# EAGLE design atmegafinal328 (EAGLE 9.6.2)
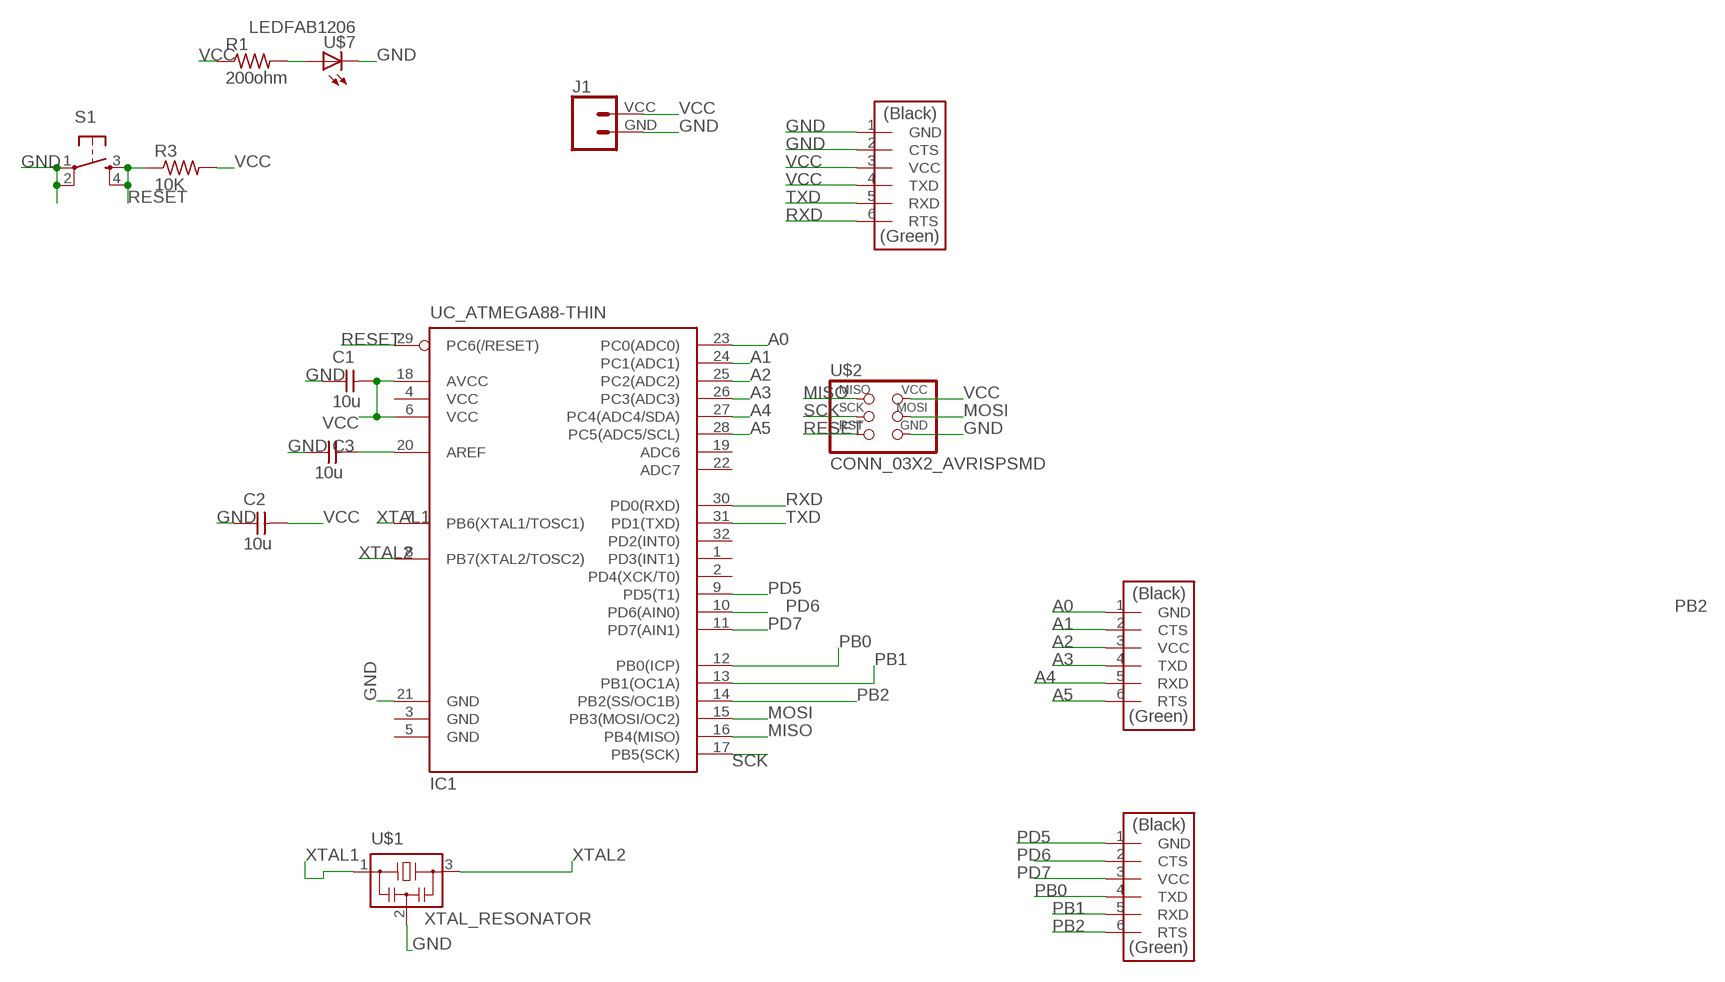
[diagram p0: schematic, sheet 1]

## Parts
C1  10u  CAP_UNPOLARIZEDFAB  [C1206FAB]
C2  10u  CAP_UNPOLARIZEDFAB  [C1206FAB]
C3  10u  CAP_UNPOLARIZEDFAB  [C1206FAB]
IC1  UC_ATMEGA88-THIN  [TQFP32-08THIN]
J1  CONN_024UCON-15767  [JST-2-SMD-VERT]
R1  200ohm  R1206FAB  [R1206FAB]
R3  10K  R1206FAB  [R1206FAB]
S1  SW_SWITCH_TACTILE_6MM6MM_SWITCH  [6MM_SWITCH]
U$1  XTAL_RESONATOR  [EFOBM]
U$2  CONN_03X2_AVRISPSMD  [2X03SMD]
U$3  CONN_06_FTDI-SMD-HEADER  [1X06SMD]
U$4  CONN_06_FTDI-SMD-HEADER  [1X06SMD]
U$6  CONN_06_FTDI-SMD-HEADER  [1X06SMD]
U$7  LEDFAB1206  [LED1206FAB]

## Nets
A0: IC1.23(PC0(ADC0)) U$4.1(GND)
A1: IC1.24(PC1(ADC1)) U$4.2(CTS)
A2: IC1.25(PC2(ADC2)) U$4.3(VCC)
A3: IC1.26(PC3(ADC3)) U$4.4(TXD)
A4: IC1.27(PC4(ADC4/SDA)) U$4.5(RXD)
A5: IC1.28(PC5(ADC5/SCL)) U$4.6(RTS)
GND: C1.1 C2.1 C3.1 IC1.21(GND) J1.GND S1.1(P) S1.2(P1) U$1.2 U$2.6(GND) U$3.1(GND) U$3.2(CTS) U$7.2(C)
MISO: IC1.16(PB4(MISO)) U$2.1(MISO)
MOSI: IC1.15(PB3(MOSI/OC2)) U$2.4(MOSI)
N$1: R1.2 U$7.1(A)
N$2: C3.2 IC1.20(AREF)
PB0: IC1.12(PB0(ICP)) U$6.4(TXD)
PB1: IC1.13(PB1(OC1A)) U$6.5(RXD)
PB2: IC1.14(PB2(SS/OC1B)) U$6.6(RTS)
PD5: IC1.9(PD5(T1)) U$6.1(GND)
PD6: IC1.10(PD6(AIN0)) U$6.2(CTS)
PD7: IC1.11(PD7(AIN1)) U$6.3(VCC)
RESET: IC1.29(PC6(/RESET)) R3.1 S1.3(S) S1.4(S1) U$2.5(RST)
RXD: IC1.30(PD0(RXD)) U$3.6(RTS)
SCK: IC1.17(PB5(SCK)) U$2.3(SCK)
TXD: IC1.31(PD1(TXD)) U$3.5(RXD)
VCC: C1.2 C2.2 IC1.6(VCC) IC1.18(AVCC) J1.VCC R1.1 R3.2 U$2.2(VCC) U$3.3(VCC) U$3.4(TXD)
XTAL1: IC1.7(PB6(XTAL1/TOSC1)) U$1.1
XTAL2: IC1.8(PB7(XTAL2/TOSC2)) U$1.3
Unconnected: IC1.1(PD3(INT1)) IC1.2(PD4(XCK/T0)) IC1.19(ADC6) IC1.22(ADC7) IC1.32(PD2(INT0))

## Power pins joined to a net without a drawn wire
GND: IC1.3(GND) IC1.5(GND)
VCC: IC1.4(VCC)

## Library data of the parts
C1-C3 = fab:CAP_UNPOLARIZED
IC1 = fab:UC_ATMEGA88-THIN
J1 = SparkFun-Connectors:CONN_02: Multi connection point. Often used as Generic Header-pin footprint for 0.1 inch spaced/style header connections
R1 R3 = fab:R: Resistor (US Symbol)
S1 = fab:SW_SWITCH_TACTILE_6MM: OMRON SWITCH
U$1 = fab:XTAL_RESONATOR
U$2 = fab:CONN_03X2_AVRISP
U$3 U$4 U$6 = fab:CONN_06_FTDI-SMD-HEADER
U$7 = fab:LED: LED

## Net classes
0 default: width 0.305 mm, drill 0.356 mm, clearance 0.305 mm

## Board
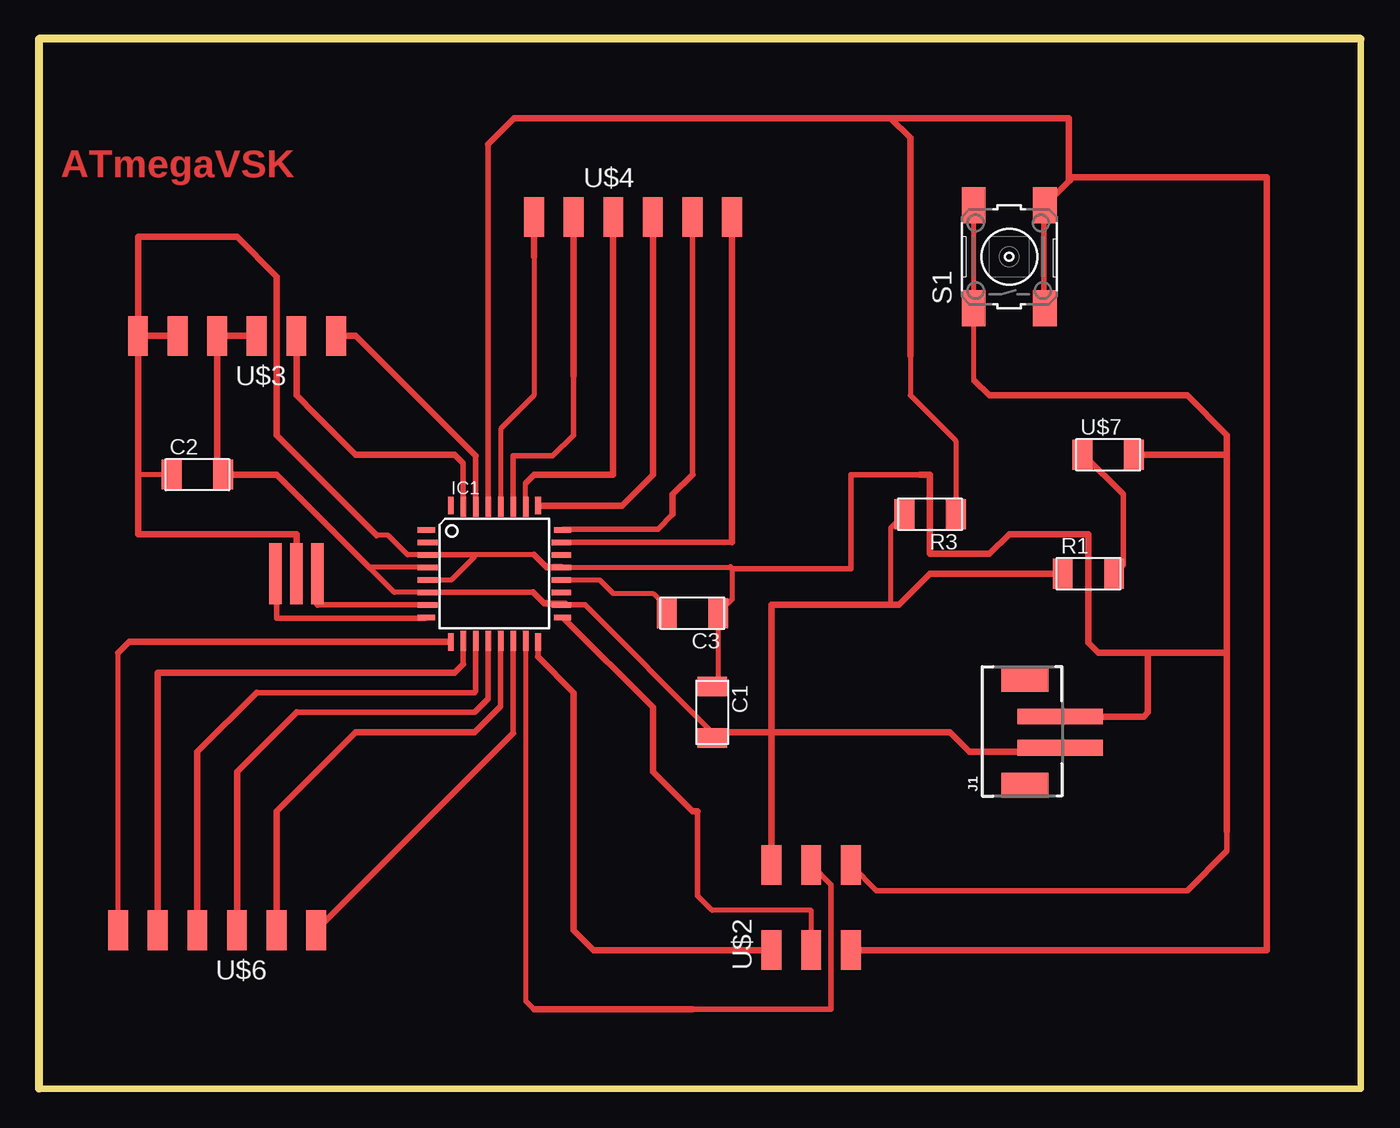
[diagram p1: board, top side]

Size 84.76 x 67.3 mm. Coordinates in mm from the lower left corner, seen from the top.
Outline: 0,67.3 0,0 84.76,0 84.76,67.3 0,67.3
Copper layers (1*16): Top 0.035mm / dielectric 1.5mm / Bottom 0.035mm
Design rules "default *": minimum track width 12mil, minimum drill 0.35mm, track to track 14mil, track to pad 14mil, pad to pad 6mil, via to via 6mil, smd to smd 6mil, copper to edge 40mil, drill to drill 6mil, minimum pad ring 10mil, minimum via ring 8mil, stop-mask expansion 4mil, vias tented up to drill 0mil, thermal gap 10mil

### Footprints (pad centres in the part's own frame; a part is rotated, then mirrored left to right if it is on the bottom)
C1206FAB = smd 1.27 x 1.905: 1 -1.651,0; 2 1.651,0
TQFP32-08THIN = smd 1.118 x 0.356: 1 -4.369,2.8; 8 -4.369,-2.8; 17 4.369,-2.8; 24 4.369,2.8 | smd 1.27 x 0.356: 2 -4.293,2; 3 -4.293,1.2; 4 -4.293,0.4; 5 -4.293,-0.4; 6 -4.293,-1.2; 7 -4.293,-2; 18 4.293,-2; 19 4.293,-1.2; 20 4.293,-0.4; 21 4.293,0.4; 22 4.293,1.2; 23 4.293,2 | smd 0.356 x 1.118: 9 -2.8,-4.369; 16 2.8,-4.369; 25 2.8,4.369; 32 -2.8,4.369 | smd 0.356 x 1.27: 10 -2,-4.293; 14 1.2,-4.293; 15 2,-4.293; 26 2,4.293; 27 1.2,4.293; 31 -2,4.293 | smd 0.35 x 1.27: 11 -1.2,-4.293; 12 -0.4,-4.293; 13 0.4,-4.293; 28 0.4,4.293; 29 -0.4,4.293; 30 -1.2,4.293
JST-2-SMD-VERT = smd 1 x 5.5: GND 1,-2; VCC -1,-2 | smd 1.6 x 3: P$1 -3.4,0.27; P$2 3.4,0.27
R1206FAB = smd 1.27 x 1.905: 1 -1.651,0; 2 1.651,0
6MM_SWITCH = smd 2.286 x 1.524: 1 -3.302,2.286; 2 3.302,2.286; 3 -3.302,-2.286; 4 3.302,-2.286
EFOBM = smd 0.8 x 3.9: 1 -1.35,0; 2 0,0; 3 1.35,0
2X03SMD = smd 2.54 x 1.27: 1 -2.54,2.54; 2 2.92,2.54; 3 -2.54,0; 4 2.92,0; 5 -2.54,-2.54; 6 2.92,-2.54
1X06SMD = smd 2.54 x 1.27: 1 0,6.35; 2 0,3.81; 3 0,1.27; 4 0,-1.27; 5 0,-3.81; 6 0,-6.35
LED1206FAB = smd 1.27 x 1.905: 1 -1.651,0; 2 1.651,0

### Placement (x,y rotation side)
C1  43.18,24.13 270 top
C2  10.16,39.37 0 top
C3  41.91,30.48 180 top
IC1  29.21,33.02 0 top
J1  63.5,22.86 90 top
R1  67.31,33.02 0 top
R3  57.15,36.83 180 top
S1  62.23,53.34 90 top
U$1  16.51,33.02 180 top
U$2  49.53,11.43 90 top
U$3  12.7,48.26 90 top
U$4  38.1,55.88 270 top
U$6  11.43,10.16 90 top
U$7  68.58,40.64 0 top

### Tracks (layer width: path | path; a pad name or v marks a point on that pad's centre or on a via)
A0
  Top 0.356: IC1.23 44.45,35.02
  Top 0.406: U$4.1 44.45,35.02
A1
  Top 0.356: IC1.24 33.66,35.88 39.69,35.88 40.64,36.83 | U$4.2 41.91,39.37
  Top 0.406: 40.64,36.83 40.64,38.1 41.91,39.37
A2
  Top 0.406: U$4.3 39.37,39.37 37.39,37.39 IC1.25
A3
  Top 0.305: IC1.26 31.21,38.83
  Top 0.356: 31.21,38.83 31.75,39.37
  Top 0.406: 31.75,39.37 36.83,39.37 U$4.4
A4
  Top 0.356: IC1.27 30.41,40.57 32.95,40.57 34.29,41.91 34.29,45.72
  Top 0.406: U$4.5 34.29,45.72
A5
  Top 0.305: U$4.6 31.7,55.68 31.7,54.69 31.75,54.61 | 31.75,53.34 31.75,44.45 29.61,42.31 IC1.28
  Top 0.406: 31.75,54.61 31.75,53.34
GND
  Top 0.305: 60.01,45.4 59.94,45.47 S1.1 S1.2 | IC1.3 23.65,34.22 22.38,35.49 21.66,35.49 | IC1.5 26.46,32.62 27.91,34.07 27.77,34.22 IC1.3 | 44.45,33.34 44.45,31.37 C3.1 43.56,26.16 C1.1 | 31.75,34.22 IC1.3 | U$2.6 53.72,12.7 | C2.1 6.35,39.37 | IC1.21 44.37,33.42
  Top 0.356: 70.17,40.64 U$7.2 | 44.45,33.34 52.07,33.34 52.07,39.37 56.52,39.37 | 53.72,12.7 73.66,12.7 76.2,15.24 76.2,16.51
  Top 0.406: 60.01,45.4 60.96,44.45 73.66,44.45 76.2,41.91 76.2,40.64 | 76.2,40.64 76.2,27.94 | 76.2,27.94 76.2,16.51 | 70.17,40.64 76.2,40.64 | 71.12,27.94 67.94,27.94 67.31,28.58 67.31,35.56 62.23,35.56 60.96,34.29 57.15,34.29 57.15,39.37 56.52,39.37 | 71.12,27.94 76.2,27.94 | U$3.1 6.35,54.61 12.7,54.61 15.24,52.07 15.24,41.91 21.66,35.49 | U$1.2 16.51,35.56 6.35,35.56 6.35,39.37 U$3.1 | 44.37,33.42 44.45,33.34 | IC1.21 32.55,33.42 31.75,34.22 | U$3.1 U$3.2 | J1.GND 70.85,23.86 71.12,24.13 71.12,27.94
MISO
  Top 0.356: IC1.16 32.01,27.68
  Top 0.406: 32.01,27.68 34.29,25.4 34.29,10.16 35.56,8.89 U$2.1
MOSI
  Top 0.305: IC1.15 31.24,28.7 31.24,5.59 31.75,5.08
  Top 0.356: 41.91,5.08 50.8,5.08 50.8,13.08 U$2.4
  Top 0.406: 41.91,5.08 31.75,5.08
N$1
  Top 0.356: R1.2 69.53,33.59 69.53,38.1 66.99,40.64 U$7.1
N$2
  Top 0.305: IC1.20 35.96,32.62 36.83,31.75 39.37,31.75 40.26,30.86 C3.2
PB0
  Top 0.356: IC1.12 28.81,25 27.94,24.13 16.51,24.13
  Top 0.406: 16.51,24.13 12.7,20.32 U$6.4
PB1
  Top 0.356: 27.94,22.86 29.61,24.53 IC1.13
  Top 0.406: 27.94,22.86 20.32,22.86 15.24,17.78 U$6.5
PB2
  Top 0.356: IC1.14 30.41,22.79
  Top 0.406: 30.41,22.79 U$6.6
PD5
  Top 0.305: U$6.1 5.08,27.94
  Top 0.406: IC1.9 5.79,28.65 5.08,27.94
PD6
  Top 0.356: IC1.10 27.21,27.21
  Top 0.406: 27.21,27.21 26.67,26.67 7.62,26.67 U$6.2
PD7
  Top 0.356: 13.97,25.4 27.94,25.4 28.01,25.47 IC1.11
  Top 0.406: U$6.3 10.16,21.59 13.97,25.4
RESET
  Top 0.305: 55.88,46.99 55.88,44.45 58.8,41.53 R3.1
  Top 0.356: S1.3 64.45,50.16 64.45,56.52 S1.4 | 28.81,60.56 IC1.29
  Top 0.406: 66.04,58.17 66.04,62.23 54.61,62.23 | 54.61,62.23 30.48,62.23 28.81,60.56 | 66.04,58.17 S1.4 | 55.88,46.99 55.88,60.96 54.61,62.23 | U$2.5 78.74,8.89 78.74,58.42 66.29,58.42 66.04,58.17
RXD
  Top 0.356: 28.01,40.57 IC1.30
  Top 0.406: 28.01,40.57 25.4,43.18 20.32,48.26 U$3.6
SCK
  Top 0.305: U$2.3 49.53,11.43 43.18,11.43 42.23,12.38
  Top 0.356: 42.23,17.78 42.23,12.38 | IC1.17 33.66,30.16
  Top 0.406: 33.66,30.16 39.37,24.45 39.37,20.32 41.91,17.78 42.23,17.78
TXD
  Top 0.356: IC1.31 27.21,40.1 26.67,40.64
  Top 0.406: 26.67,40.64 20.32,40.64 17.78,43.18 16.51,44.45 U$3.5
VCC
  Top 0.305: R3.2 54.61,35.94 54.61,31.02 | IC1.4 21.19,33.42 22.79,31.82 IC1.6 | C1.2 43.18,22.86 35.02,31.02 | 11.43,39.75 C2.2
  Top 0.356: IC1.6 31.68,31.82 | 35.02,31.02 33.83,31.02
  Top 0.406: 21.19,33.42 15.24,39.37 C2.2 | U$2.2 46.99,22.86 | 46.99,22.86 46.99,31.02 54.61,31.02 55.15,31.02 57.15,33.02 R1.1 | 11.43,39.75 U$3.3 U$3.4 | 31.68,31.82 32.38,31.12 32.6,31.12 32.64,31.08 33.75,31.08 33.79,31.05 | 33.83,31.02 33.79,31.05 | 33.79,31.05 33.61,31.02 IC1.18 | C1.2 43.56,22.86 46.99,22.86 | 46.99,22.86 58.42,22.86 59.69,21.59 65.23,21.59 J1.VCC
XTAL1
  Top 0.356: IC1.7 17.86,31.02
  Top 0.406: 17.86,31.02 U$1.1
XTAL2
  Top 0.356: IC1.8 24.77,30.16 15.24,30.16 15.24,33.02 U$1.3

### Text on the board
Top: ATmegaVSK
